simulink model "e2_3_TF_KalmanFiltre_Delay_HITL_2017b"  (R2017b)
settings: Solver=ode4  StartTime=0.0  StopTime=100  FixedStep=sampleTime  RelTol=1e-3  EnableMultiTasking=on
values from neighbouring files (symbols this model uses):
  k_d_x = 0.7    [startSimulation.m]
  k_d_y = 0.7    [startSimulation.m]
  k_d_yaw = 0.05    [startSimulation.m]
  k_d_z = 0.05    [startSimulation.m]
  k_i_x = 0.01    [startSimulation.m]
  k_i_y = 0.01    [startSimulation.m]
  k_i_yaw = 0.01    [startSimulation.m]
  k_i_z = 0.01    [startSimulation.m]
  k_p_x = 1    [startSimulation.m]
  k_p_y = 1    [startSimulation.m]
  k_p_yaw = 2    [startSimulation.m]
  k_p_z = 3    [startSimulation.m]
  saturation_psi = 2    [startSimulation.m]
  saturation_x = 2    [startSimulation.m]
  saturation_y = 2    [startSimulation.m]
  saturation_z = 2    [startSimulation.m]
undefined symbols (not defined in the file or in its folder): DiscIntNeverNeededParam, KiRollAttitude, sigbuilder_block
libraries: simulink x10, aerolibanimutils x2, etargetslib x2
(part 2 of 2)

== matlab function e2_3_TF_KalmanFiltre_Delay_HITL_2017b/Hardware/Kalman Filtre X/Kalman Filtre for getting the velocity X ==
function [Covariance_matrice,X_Kalmanfiltred] = fcn(Mesurement_Velocity) % Mesurement_State

% Persistent process for saving the last state and initilizing the variable
persistent P0_static;
if isempty(P0_static)
    P0_static=[[0.1,0 0;0,0.1,0;0 0 0.1] zeros(3) zeros(3) ;zeros(3) [0.1,0 0;0,0.1,0;0 0 0.1] zeros(3);zeros(3) zeros(3) [0.1,0 0;0,0.1,0;0 0 0.1]]; % the initilized matrice of estimated error
end

persistent Xkf_static;
if isempty(Xkf_static)
    Xkf_static=[0;0;0;0;0;0;0;0;0]; % the initilized state from Kalman Estimaton
end

% Determine the constants

% Simple time
Ts =1/25;

% Process Noise
p_var =0.05; % sigma
Q = eye(3)*p_var^2; % the covariance matrice of process noise
W=Q*randn(3,1);  % process noise
Q_delay=[Q zeros(3) zeros(3);zeros(3) Q zeros(3);zeros(3) zeros(3) Q];
% Mesurement Noise
m_var = 0.01; % sigma
R = [m_var^2 ];  % the covariance matrice of mesurement noise
V=R*randn; % mesurement noise
R_delay=R;
V_delay=R_delay*randn;
% Observation matrice
H=[1 0 0];
H_delay=[0 0 0 0 0 0 H];
% The indentity matrice
I=eye(3); 
I_delay=eye(9);

A=[1 Ts 0.5*(Ts^2);0 1 Ts;0 0 1];
A_delay=[A zeros(3) zeros(3);zeros(3) A zeros(3); zeros(3) zeros(3) A];
% Steady-State equation

% persistent X_real_static;
% if isempty(X_real_static)
%     X_real_static=[0;0]; % the initilized state from Kalman Estimaton
% end
% X_real_forward=X_real_static;
% X_real=A*X_real_forward+W;
% X_real_static=X_real;    
% Mesurement_Velocity=H_delay*(Mesurement_State)+V_delay;

%   Kalman Update process
    X_pre=A_delay*Xkf_static; % State estimation
    P_pre=A_delay*P0_static*A_delay'+Q_delay; % Covariance matrice estimation

    Kg=P_pre*H_delay'*inv(H_delay*P_pre*H_delay'+R_delay); % Kalman Gain calculation

    X_Kalmanfiltred=X_pre+Kg*(Mesurement_Velocity-H_delay*X_pre); % State estimation update
    Covariance_matrice=(I_delay-Kg*H_delay)*P_pre; % Covariance matrice estimation update

% update the value of the persistent variable for iterating the Kalman process
P0_static=Covariance_matrice;
Xkf_static=X_Kalmanfiltred;

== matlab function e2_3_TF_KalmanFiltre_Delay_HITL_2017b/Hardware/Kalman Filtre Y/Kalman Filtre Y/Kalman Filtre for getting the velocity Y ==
function [Covariance_matrice,X_Kalmanfiltred] = fcn(Mesurement_Velocity)

% Persistent process for saving the last state and initilizing the variable
persistent P0_static;
if isempty(P0_static)
    P0_static=[0.1,0 0;0,0.1,0;0 0 0.1]; % the initilized matrice of estimated error
end

persistent Xkf_static;
if isempty(Xkf_static)
    Xkf_static=[0;0;0]; % the initilized state from Kalman Estimaton
end

% Determine the constants

% Simple time
Ts =1/25;

% Process Noise
p_var =0.05; % sigma
Q = eye(3)*p_var^2; % the covariance matrice of process noise
W=Q*randn(3,1);  % process noise

% Mesurement Noise
m_var =0.01; % sigma
R = [m_var^2 ];  % the covariance matrice of mesurement noise
V=R*randn; % mesurement noise

% Observation matrice
H=[1 0 0];

% The indentity matrice
I=eye(3); 

% State Transition Martrix
A=[1 Ts 0.5*(Ts^2);0 1 Ts;0 0 1];

% Steady-State equation

% persistent X_real_static;
% if isempty(X_real_static)
%     X_real_static=[0;0]; % the initilized state from Kalman Estimaton
% end
% X_real_forward=X_real_static;
% X_real=A*X_real_forward+W;
% Mesurement_Velocity=H*(X_real)+V;
% X_real_static=X_real;    

%   Kalman Update process
    X_pre=A*Xkf_static; % State estimation
    P_pre=A*P0_static*A'+Q; % Covariance matrice estimation

    Kg=P_pre*H'*inv(H*P_pre*H'+R); % Kalman Gain calculation

    X_Kalmanfiltred=X_pre+Kg*(Mesurement_Velocity-H*X_pre); % State estimation update
    Covariance_matrice=(I-Kg*H)*P_pre; % Covariance matrice estimation update

% update the value of the persistent variable for iterating the Kalman process
P0_static=Covariance_matrice;
Xkf_static=X_Kalmanfiltred;

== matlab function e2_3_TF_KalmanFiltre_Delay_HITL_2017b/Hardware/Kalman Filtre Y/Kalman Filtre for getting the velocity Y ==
function [Covariance_matrice,X_Kalmanfiltred] = fcn(Mesurement_Velocity) % Mesurement_State

% Persistent process for saving the last state and initilizing the variable
persistent P0_static;
if isempty(P0_static)
       P0_static=[[0.1,0 0;0,0.1,0;0 0 0.1] zeros(3) zeros(3) ;zeros(3) [0.1,0 0;0,0.1,0;0 0 0.1] zeros(3);zeros(3) zeros(3) [0.1,0 0;0,0.1,0;0 0 0.1]]; % the initilized matrice of estimated error 
end

persistent Xkf_static;
if isempty(Xkf_static)
    Xkf_static=[0;0;0;0;0;0;0;0;0]; % the initilized state from Kalman Estimaton
end

% Determine the constants

% Simple time
Ts =1/25;

% Process Noise
p_var =0.05; % sigma
Q = eye(3)*p_var^2; % the covariance matrice of process noise
W=Q*randn(3,1);  % process noise
Q_delay=[Q zeros(3) zeros(3);zeros(3) Q zeros(3);zeros(3) zeros(3) Q];
% Mesurement Noise
m_var = 0.01; % sigma
R = [m_var^2 ];  % the covariance matrice of mesurement noise
V=R*randn; % mesurement noise
R_delay=R;
V_delay=R_delay*randn;
% Observation matrice
H=[1 0 0];
H_delay=[0 0 0 0 0 0 H];
% The indentity matrice
I=eye(3); 
I_delay=eye(9);

A=[1 Ts 0.5*(Ts^2);0 1 Ts;0 0 1];
A_delay=[A zeros(3) zeros(3);zeros(3) A zeros(3); zeros(3) zeros(3) A];
% Steady-State equation

% persistent X_real_static;
% if isempty(X_real_static)
%     X_real_static=[0;0]; % the initilized state from Kalman Estimaton
% end
% X_real_forward=X_real_static;
% X_real=A*X_real_forward+W;
% X_real_static=X_real;    
% Mesurement_Velocity=H_delay*(Mesurement_State)+V_delay;

%   Kalman Update process
    X_pre=A_delay*Xkf_static; % State estimation
    P_pre=A_delay*P0_static*A_delay'+Q_delay; % Covariance matrice estimation

    Kg=P_pre*H_delay'*inv(H_delay*P_pre*H_delay'+R_delay); % Kalman Gain calculation

    X_Kalmanfiltred=X_pre+Kg*(Mesurement_Velocity-H_delay*X_pre); % State estimation update
    Covariance_matrice=(I_delay-Kg*H_delay)*P_pre; % Covariance matrice estimation update

% update the value of the persistent variable for iterating the Kalman process
P0_static=Covariance_matrice;
Xkf_static=X_Kalmanfiltred;
